//FC650	Copy
// ***************************************************************************
FUNCTION "FC_COPY" : VOID

TITLE =Send/Receive Empfang

AUTHOR: 	SIEMENS
FAMILY: 	SISTARS7
VERSION: 	4.02

//KNOW_HOW_PROTECT

// Datum	 Name			Aktion
// ---------------------------------------------------------------------------
// 19.05.99  Mahler		Neu



//Eingabeparameter
VAR_INPUT
	iQDB		: INT;		//Aufrufmodus	Quell-Datenbausteinnr. 1 - 64 000
	iQDW		: INT;		//		      Quell-Datenwort. 0 - 64 000
	bQTYP		: BYTE;		//			Quell-Typ  z.B.: 84=DB 85=DI 83=Merker 8C=VAR_TEMP
	iZDB		: INT;		//Aufrufmodus     Ziel
	iZDW		: INT;		//
	bZTyp		: BYTE;		//
END_VAR

//Eingabe - Ausgabeparameter
VAR_IN_OUT
	iLenByte	: INT;            //Laenge in Byte wenn =0 nach Ausfuehrung dh. Fehler
END_VAR


//Temporäre/Lokale Variable
VAR_TEMP

	anyQUEL	: ANY; 	         //Offset=0, Zeiger muss an erster Stelle stehen
	anyZIEL	: ANY;		   //Offset=10,
	iret		: INT;

END_VAR

BEGIN

NETWORK
TITLE = Vorbesetzen der Zeiger
// ===========================================================================
//Pionter fuer den Empfangspuffer zusammenstellen
//Any-Pointer:
//Byte 0	: S7-Typ 		= 16=10H                 LB0,LB10
//Byte 1	: Datentyp		= 02=Byte			 LB1,LB11
//Byte 2/3	: Wiederholungsfaktor				 LW2,LW12
//Byte 4/5	: DB-Nummer						 LW4,LW14
//Byte 6-9	: Bereichszeiger					 LD6,LD16

	L 16;		//S7-Typ
	T LB 0;
	T LB 10;
	L 2;		//Datentyp=Byte
	T LB1;
	T LB11;

	L iLENByte;		//Anzahl
	T LW  2;
	T LW 12;

     L iQDB;		//DB-NR
	T LW 4;
      L iZDB;		//DB-NR
	T LW 14;

	L iQDW;
	SLD 3;
	T LD 6;

	L iZDW;
	SLD 3;
	T LD 16;

	L bQTyp;
	T LB  6;		//Kennung DB=84 oder VAR_TEMP=8C
	L bZTyp;
	T LB 16;		//Kennung DB=84 oder VAR_TEMP=8C


	CALL "BLKMOV" (
			SRCBLK 	:= #anyQUEL,
			RET_VAL	:= #iret,
			DSTBLK	:= #anyZIEL
			  );

	L #iret;
	l 0;
	==I;
 	spb end1;
	T  iLENByte;

end1: NOP 0;


END_FUNCTION
